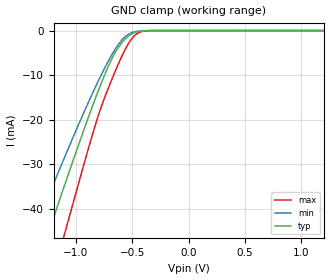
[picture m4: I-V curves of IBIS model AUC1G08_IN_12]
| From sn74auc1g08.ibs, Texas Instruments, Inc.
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[Model]   AUC1G08_IN_12
Model_type  Input
Vinl=0.385
Vinh=0.845
| variable   typ   min   max
C_comp   2.36pF   2.03pF   2.74pF
[Temperature Range]   40   100   -40
| Ambient temperature   25   85   -40
[Voltage range]   1.2   1.1   1.3
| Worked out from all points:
|   GND clamp passes 1 mA (typ) near -0.52 V on its own axis
[GND Clamp]
| AUC1G08_IN_12
|   Voltage   I(typ)   I(min)   I(max)
-3.6V     -228.2mA   -191.9mA   -274.5mA
-1.395V   -56.72mA   -46.45mA   -72.64mA
-1.345V   -52.92mA   -43.33mA   -68.03mA
-1.255V   -46.12mA   -37.74mA   -59.72mA
-1.215V   -43.11mA   -35.29mA   -56.03mA
-1.09V    -33.82mA   -27.72mA   -44.53mA
-835mV    -15.66mA   -13.06mA   -21.7mA
-700mV    -7.266mA   -6.224mA   -12.08mA
-580mV    -2.329mA   -1.757mA   -5.052mA
-465mV    -313.5uA   -199.6uA   -806.3uA
-330mV    -7.615uA   -7.137uA   -10.28uA
1.2V      207.9pA    721.7pA    28.54pA
